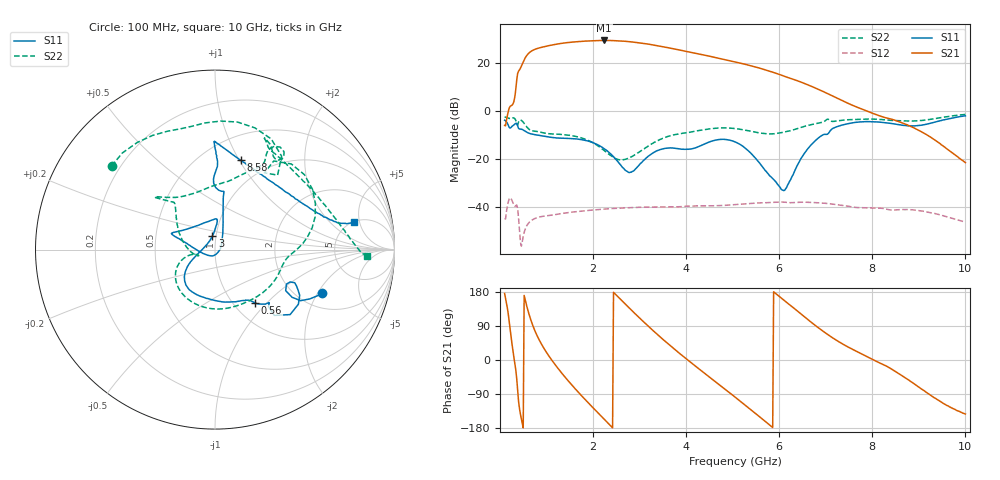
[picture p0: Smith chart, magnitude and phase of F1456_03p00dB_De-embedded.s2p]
! Integrated Device Technology
! Corporate Headquarters
! 6024 Silver Creek Valley Road
! San Jose, CA 95138  USA
! Phone:  1-408-284-8200
! Toll Free:  1-800-223-1366
! Webpage:  http://www.idt.com/
! Timing and RF Division
! 515 Groton Road, Suite 102
! Westford, MA 01886-6024
! Device:  F1456
! Description: 6-bit 0.5 dB Transmit Variable Gain Amplifier
! Frequency:  2100.0 -  2950.00 MHz
! Package:  6x6 mm Thin QFN Plastic Package: 28 pin
! State:  6
! Atten State:  3.0 dB
! Voltage:  +5.00 Volts
! Current:  214.757 mA
! Data:  The device was measured on a the F1455 evaluation board which has
!  individual transmission lines to the RF pins.  Data was collected
!  using a calibrated network analyzer.  The evaluation board was
!  de-embedded using a TRL calibration technique.
!  The reference plane is the edge of the package pin.
!  Pin  1 = CSb
!  Pin  2 = DATA
!  Pin  3 = CLK
!  Pin  4 = RSET
!  Pin  5 = GND
!  Pin  6 = RFIN  = Port 1
!  Pin  7 = GND
!  Pin  8 = NC
!  Pin  9 = NC
!  Pin 10 = NC
!  Pin 11 = NC
!  Pin 12 = NC
!  Pin 13 = NC
!  Pin 14 = /STBY
!  Pin 15 = GND
!  Pin 16 = RFOUT  = Port 2
!  Pin 17 = GND
!  Pin 18 = NC
!  Pin 19 = NC
!  Pin 20 = NC
!  Pin 21 = GND
!  Pin 22 = NC
!  Pin 23 = GND
!  Pin 24 = NC
!  Pin 25 = NC
!  Pin 26 = NC
!  Pin 27 = GND
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# GHz S dB R 50
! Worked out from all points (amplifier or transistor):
!   496 points, 100 MHz to 10 GHz, reference 50 ohm
!   highest |S21| = 29.2 dB at 2.24 GHz (marker M1)
!   |S21| within 3 dB of that: 862.1 MHz to 3.611 GHz (2.749 GHz wide, 123 % of centre)
!   unconditionally stable (mu >= 1): start of sweep to end of sweep
!   at 1.74 GHz: K = 2.04, MAG = 29.4 dB, |S12| = -41.5 dB
!   at 5.06 GHz: K = 3.42, MAG = 21.3 dB, |S12| = -38.8 dB
!   at 10 GHz: K = 126.45, MAG = -11.7 dB, |S12| = -46.1 dB
!   S11 on the Smith chart (normalised r, x): 100 MHz: 2.65, -2.19; 560 MHz: 1.25, -0.86; 3 GHz: 0.96, +0.15; 8.58 GHz: 0.74, +1.01; 10 GHz: 5.02, +4.21
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0.1  -3.82 -22.0  -5.99 175.6  -44.57 42.4  -2.61 141.1
0.34  -5.11 -33.2  8.92 -25.8  -39.30 -142.3  -3.89 54.5
0.42  -7.47 -44.4  17.05 -128.5  -49.50 136.3  -3.89 48.3
0.56  -8.62 -53.1  22.56 149.9  -48.15 -172.5  -6.18 4.0
0.66  -9.46 -56.9  24.61 107.0  -45.61 156.1  -7.97 -7.8
0.76  -9.86 -62.1  25.61 74.6  -44.49 130.0  -8.41 -20.3
0.94  -10.44 -76.3  26.59 31.7  -43.60 95.6  -9.10 -48.3
1.12  -10.98 -91.1  27.34 -1.4  -43.16 73.2  -9.52 -74.0
1.46  -11.38 -113.8  28.36 -54.1  -42.13 43.9  -10.00 -116.4
1.76  -11.91 -130.0  28.86 -95.2  -41.47 23.3  -11.21 -142.8
2.24  -15.63 -151.1  29.22 -156.4  -40.65 -4.5  -16.37 -167.2
2.58  -22.12 -175.2  29.03 161.3  -40.25 -22.8  -20.27 -160.7
3  -22.19 101.1  28.22 110.8  -39.92 -44.2  -16.94 -178.1
3.4  -16.32 85.6  27.00 65.4  -39.81 -63.5  -12.21 148.0
4.02  -15.85 113.0  24.61 1.5  -39.45 -89.9  -9.00 131.5
4.52  -12.69 154.2  22.62 -47.2  -39.31 -112.2  -7.36 138.2
5.06  -12.87 162.3  20.29 -98.6  -38.82 -134.7  -7.31 137.0
5.7  -24.69 -152.1  17.05 -162.1  -38.03 -168.7  -9.40 116.3
6.7  -13.75 77.5  10.15 98.4  -37.89 129.0  -5.62 62.0
8.36  -5.05 83.4  -3.15 -19.9  -40.93 54.2  -3.84 62.5
8.58  -5.72 74.0  -4.49 -36.7  -40.89 48.9  -4.05 56.7
10  -2.02 11.4  -21.40 -142.5  -46.08 -26.6  -1.46 -2.5
